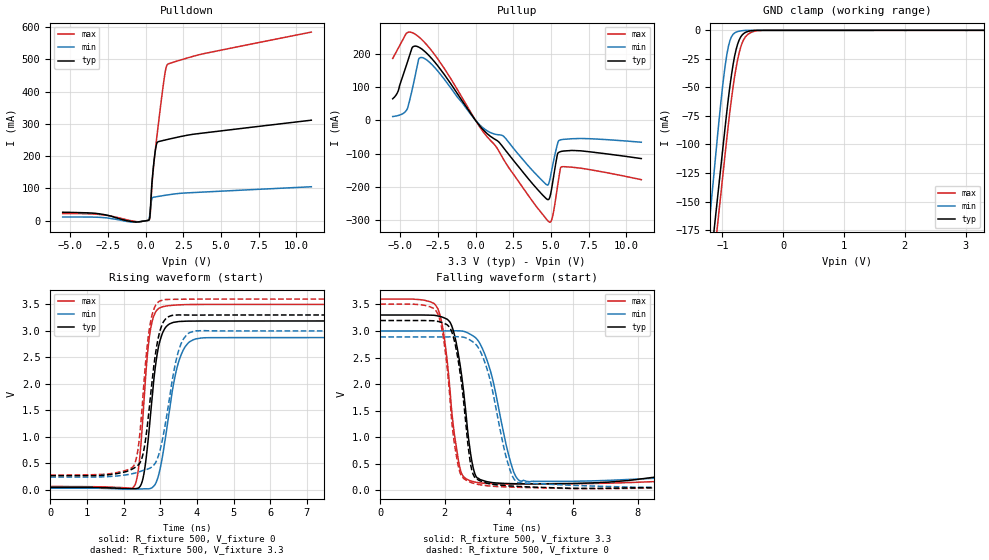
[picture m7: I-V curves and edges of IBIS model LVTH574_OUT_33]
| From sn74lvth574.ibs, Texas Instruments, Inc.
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[Model]   LVTH574_OUT_33
Model_type  3-state
Enable   Active-Low
Vref =   0
Rref =   500
Cref =   50p
Vmeas =   1.5
| variable   typ   min   max
C_comp   5.67pF   4.62pF   7.97pF
| C_pullup   4.92pF   0.29pF   7.04pF
| C_pulldown   9.54pF   2.17pF   32.43pF
| C_tri-state   5.67pF   4.62pF   7.97pF
[Temperature Range]   40   -40   100
| Ambient temperature   25   -40   85
[Voltage range]   3.3   3   3.6
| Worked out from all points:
|   slope of the pulldown table from 0 to 0.495 V, typ, clamps not added: 3.18 ohm
|   slope of the pullup table from 0 to 0.495 V, typ, clamps not added: 17.9 ohm
|   GND clamp passes 1 mA (typ) near -0.58 V on its own axis
|   rising waveform, R_fixture 500, V_fixture 0: 20-80 % time 287ps typ, 405ps min, 231ps max; typ from 0.041 V to 3.19 V
|   falling waveform, R_fixture 500, V_fixture 3.3: 20-80 % time 378ps typ, 622ps min, 359ps max; typ from 3.3 V to 0.263 V
|   rising waveform, R_fixture 500, V_fixture 3.3: 20-80 % time 316ps typ, 424ps min, 257ps max; typ from 0.261 V to 3.3 V
|   falling waveform, R_fixture 500, V_fixture 0: 20-80 % time 377ps typ, 624ps min, 364ps max; typ from 3.2 V to 0.042 V
[GND Clamp]
| LVTH574_OUT_33
|   Voltage   I(typ)   I(min)   I(max)
-5.5V     -2.862A    -3.036A    -2.891A
-1.24V    -226.5mA   -182.9mA   -251.6mA
-1.21V    -211.4mA   -165.7mA   -236.1mA
-1.17V    -191.4mA   -142.9mA   -215.7mA
-1.075V   -144mA     -89.2mA    -167.9mA
-975mV    -94.37mA   -39.09mA   -118.1mA
-925mV    -69.94mA   -20.46mA   -93.26mA
-875mV    -48.14mA   -8.719mA   -70.1mA
-800mV    -22.75mA   -2.299mA   -40.62mA
-725mV    -8.466mA   -746.4uA   -19.77mA
-575mV    -873.9uA   -11.47uA   -3.261mA
3.3V      32.83pA    25.31pA    1.683nA
[Pulldown]
| LVTH574_OUT_33
|   Voltage   I(typ)   I(min)   I(max)
-5.5V     26.14mA    11.41mA    22.29mA
-3.14V    21.76mA    10.56mA    19.6mA
-710mV    -3.659mA   -4.637mA   -2.131mA
245mV     3.449mA    8.005mA    3.326mA
315mV     33.12mA    35.95mA    22.67mA
425mV     118.9mA    68.07mA    110mA
580mV     192.7mA    73.06mA    190.3mA
710mV     233.6mA    74.11mA    244.7mA
1.245V    249.3mA    78.23mA    443.5mA
1.365V    250.6mA    79.1mA     474.6mA
1.47V     251.7mA    79.85mA    484.5mA
11V       311.3mA    105.1mA    584.1mA
[Pullup]
| LVTH574_OUT_33
|   Voltage   I(typ)   I(min)   I(max)
-5.5V     64.85mA    11.59mA    185.8mA
-4.6V     164.3mA    29.39mA    261.2mA
-4.205V   218.5mA    92.94mA    263.2mA
-3.775V   219.9mA    183.8mA    250.7mA
-3.465V   210.4mA    187.3mA    237.6mA
270mV     -15.96mA   -13.16mA   -19.22mA
1.85V     -81.89mA   -47.23mA   -116.3mA
4.895V    -234.1mA   -183.8mA   -304.9mA
5.115V    -186.5mA   -135mA     -287.6mA
5.435V    -101.1mA   -70.96mA   -199.1mA
5.69V     -93mA      -57.8mA    -139.6mA
11V       -114.5mA   -65.47mA   -177.8mA
[Ramp]
| LVTH574_OUT_33
| variable   typ   min   max
dV/dt_r   1.90/2.91E-10   1.72/4.14E-10   2.09/2.34E-10
dV/dt_f   1.91/3.99E-10   1.70/6.43E-10   2.09/3.84E-10
R_load = 500
[Rising Waveform]
| LVTH574_OUT_33
R_fixture =   500
C_fixture =   0
L_fixture =   0
V_fixture =   0
V_fixture_min = 0
V_fixture_max = 0
|   Time   V(typ)   V(min)   V(max)
0s        41.42mV    24.68mV    57.22mV
2.295ns   16.76mV    7.001mV    68.68mV
2.42ns    36.56mV    9.192mV    468.4mV
2.54ns    246mV      12.92mV    1.506V
2.745ns   1.49V      22.85mV    3.069V
2.95ns    2.69V      259.4mV    3.418V
3.225ns   3.118V     1.372V     3.475V
3.6ns     3.178V     2.596V     3.493V
4.19ns    3.185V     2.868V     3.498V
50ns      3.188V     2.873V     3.5V
[Falling Waveform]
| LVTH574_OUT_33
R_fixture =   500
C_fixture =   0
L_fixture =   0
V_fixture =   3.3
V_fixture_min = 3
V_fixture_max = 3.6
|   Time   V(typ)   V(min)   V(max)
0s        3.3V       3V         3.6V
1.72ns    3.291V     3.001V     3.485V
1.95ns    3.256V     3.001V     3.026V
2.17ns    3.162V     3.002V     1.865V
2.51ns    2.243V     3V         346.7mV
2.855ns   522.4mV    2.918V     171.9mV
3.165ns   193.3mV    2.682V     139mV
4.055ns   129.1mV    523.2mV    121.5mV
4.37ns    125.5mV    177.2mV    121.4mV
50ns      263.4mV    233.6mV    273mV
[Rising Waveform]
| LVTH574_OUT_33
R_fixture =   500
C_fixture =   0
L_fixture =   0
V_fixture =   3.3
V_fixture_min = 3
V_fixture_max = 3.6
|   Time   V(typ)   V(min)   V(max)
0s        260.8mV    234.8mV    273.4mV
2.28ns    403.7mV    305.7mV    451.7mV
2.405ns   466.2mV    330.3mV    819.7mV
2.53ns    672.4mV    359.8mV    1.783V
2.735ns   1.777V     410.6mV    3.168V
2.925ns   2.794V     588.6mV    3.527V
3.13ns    3.21V      1.206V     3.591V
3.515ns   3.3V       2.654V     3.596V
3.985ns   3.297V     3.001V     3.599V
50ns      3.3V       3V         3.6V
[Falling Waveform]
| LVTH574_OUT_33
R_fixture =   500
C_fixture =   0
L_fixture =   0
V_fixture =   0
V_fixture_min = 0
V_fixture_max = 0
|   Time   V(typ)   V(min)   V(max)
0s        3.196V     2.888V     3.505V
1.72ns    3.187V     2.888V     3.389V
1.95ns    3.152V     2.889V     2.917V
2.165ns   3.06V      2.889V     1.738V
2.495ns   2.153V     2.89V      309.7mV
2.84ns    395.8mV    2.81V      145.5mV
3.295ns   140.5mV    2.329V     90.47mV
3.94ns    88.55mV    565.8mV    66.05mV
4.3ns     75.58mV    145.7mV    59.55mV
50ns      41.7mV     24.6mV     57.3mV
